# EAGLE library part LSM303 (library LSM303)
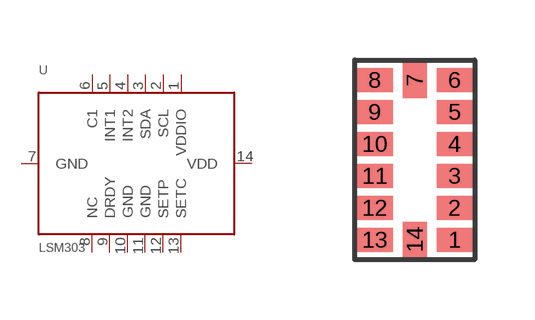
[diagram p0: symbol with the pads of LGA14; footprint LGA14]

Designator prefix -

## LSM303  [LGA14]
1  VDDIO  pwr
2  SCL
3  SDA
4  INT2  out
5  INT1  out
6  C1
7  GND  pwr
8  NC
9  DRDY  out
10  GND  pwr
11  GND  pwr
12  SETP
13  SETC
14  VDD  pwr

## Footprint LGA14 (pad centres in mm)
smd 0.9 x 0.6: 1 1,-2; 2 1,-1.2; 3 1,-0.4; 4 1,0.4; 5 1,1.2; 6 1,2; 8 -1,2; 9 -1,1.2; 10 -1,0.4; 11 -1,-0.4; 12 -1,-1.2; 13 -1,-2
smd 0.6 x 0.9: 7 0,2; 14 0,-2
